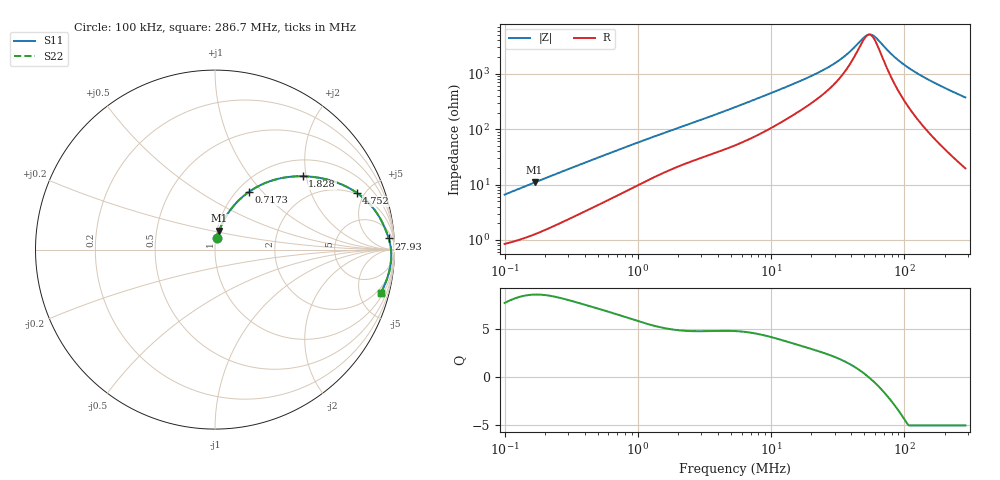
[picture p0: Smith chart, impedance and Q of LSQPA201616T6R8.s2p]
! LSQPA201616T6R8  S-PARAMETER MODEL  ( General Type )
! Model Generated by TAIYO YUDEN Corporation (http://www.ty-top.com)
! Version 2.0
! TAIYO YUDEN Control No. 100810NF25SB-FKC
! Copyright(c) 2007 TAIYO YUDEN CO.,LTD. All Rights Reserved.
! Product Description (link to TY-COMPAS)
! https://ds.yuden.co.jp/TYCOMPAS/or/detail?pn=LSQPA201616T6R8M&u=M
! Products Name : Inductors
! Characteristics :
!  Inductance : 6.8 uH , SRF(min) : 38 MHz , DC Resistance(max) : 0.767 Ohm
!  Rated Current : Saturation :450 mA , Temp Rise : 450 mA (40 degC)
!  Case Size : 2.0 x 1.6 / 0.079 x 0.063 [mm/inch] , Thickness : 1.6 / 0.063 [mm/inch]
!  (Conditions: Temperature = 25 degC , DC Bias Current/Voltage = 0A / 0V)
! External Node Assignments :
!  1  o---GGG---o  2
! GND o---------o GND
! Frequency Range : 0.1MHz  -  286.687601MHz  [ 402 STEP ]
# MHz S RI R 50
! Freq[MHz].  S11 Real  S11 Imag  S21 Real  S21 Imag  S12 Real  S12 Imag  S22 Real  S22 Imag
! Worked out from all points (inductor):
!   401 points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, 100 kHz to 286.7 MHz, reference 50 ohm
!   read as one part in series: L = 10.4 uH near 104.1 kHz
!   highest Q = 8.56 at 167.8 kHz (marker M1), where L = 10.3 uH
!   self-resonance near 53.99 MHz
!   S11 on the Smith chart (normalised r, x): 100 kHz: 1.02, +0.13; 717.3 kHz: 1.13, +0.84; 1.828 MHz: 1.39, +1.91; 4.752 MHz: 1.91, +4.38; 27.93 MHz: 12, +25; 286.7 MHz: 1.39, -7.47
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0.1  0.0126 0.0641  0.9874 -0.0641  0.9874 -0.0641  0.0126 0.0641
0.167777  0.0237 0.1046  0.9763 -0.1046  0.9763 -0.1046  0.0237 0.1046
0.379416  0.0777 0.21  0.9223 -0.21  0.9223 -0.21  0.0777 0.21
0.717313  0.188 0.3209  0.812 -0.3209  0.812 -0.3209  0.188 0.3209
1.439567  0.4037 0.404  0.5963 -0.404  0.5963 -0.404  0.4037 0.404
1.827908  0.4888 0.4088  0.5112 -0.4088  0.5112 -0.4088  0.4888 0.4088
2.889051  0.6461 0.3846  0.3539 -0.3846  0.3539 -0.3846  0.6461 0.3846
4.751638  0.7892 0.3168  0.2108 -0.3168  0.2108 -0.3168  0.7892 0.3168
5.354322  0.8166 0.2963  0.1834 -0.2963  0.1834 -0.2963  0.8166 0.2963
9.536008  0.9072 0.1951  0.0928 -0.1951  0.0928 -0.1951  0.9072 0.1951
20.31517  0.9568 0.0942  0.0432 -0.0942  0.0432 -0.0942  0.9568 0.0942
27.93295  0.9678 0.0619  0.0322 -0.0619  0.0322 -0.0619  0.9678 0.0619
36.18117  0.9744 0.0375  0.0256 -0.0375  0.0256 -0.0375  0.9744 0.0375
49.74838  0.9798 0.00779  0.0202 -0.00779  0.0202 -0.00779  0.9798 0.00779
53.87075  0.9807 0.000212  0.0193 -0.000212  0.0193 -0.000212  0.9807 0.000212
57.1852  0.9813 -0.00555  0.0187 0.00555  0.0187 0.00555  0.9813 -0.00555
60.70356  0.9817 -0.0114  0.0183 0.0114  0.0183 0.0114  0.9817 -0.0114
77.07906  0.9822 -0.0358  0.0178 0.0358  0.0178 0.0358  0.9822 -0.0358
97.87206  0.9807 -0.0626  0.0193 0.0626  0.0193 0.0626  0.9807 -0.0626
129.3207  0.9756 -0.0984  0.0244 0.0984  0.0244 0.0984  0.9756 -0.0984
188.7535  0.9601 -0.158  0.0399 0.158  0.0399 0.158  0.9601 -0.158
286.6876  0.9222 -0.2428  0.0778 0.2428  0.0778 0.2428  0.9222 -0.2428
